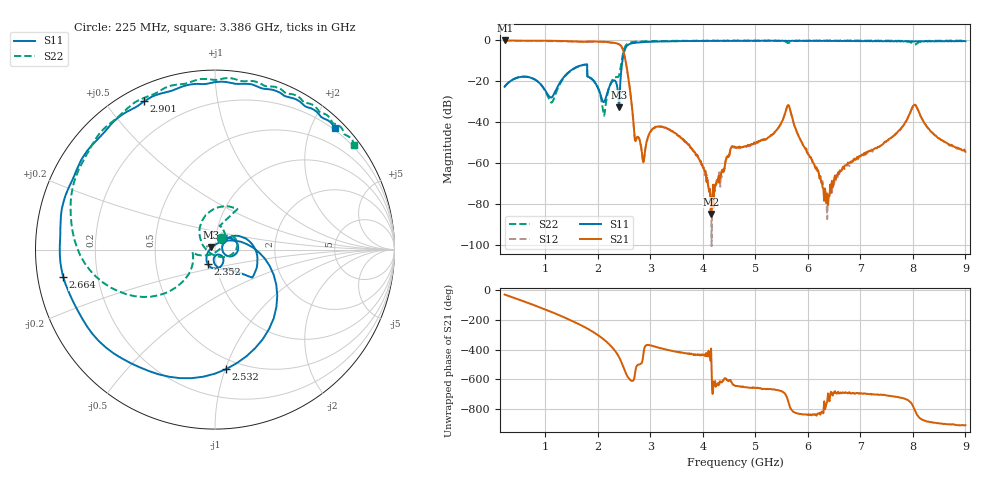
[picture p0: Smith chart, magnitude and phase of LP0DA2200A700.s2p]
!Agilent Technologies,E8358A,US41080443,A.07.50.56
!Agilent E8358A: A.07.50.56
!Date: Monday, May 09, 2016 11:42:41
!Correction: S11(Full 2 Port(1,2))
!S21(Full 2 Port(1,2))
!S12(Full 2 Port(1,2))
!S22(Full 2 Port(1,2))
!S2P File: Measurements: S11, S21, S12, S22:Log Frequency Sweep
# Hz S  dB  R 50
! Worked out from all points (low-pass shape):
!   1601 points, 225 MHz to 9 GHz, reference 50 ohm
!   highest |S21| = 0.00 dB at 226 MHz (marker M1); lowest = -85.0 dB at 4.157 GHz (marker M2)
!   |S21| within 3 dB of the highest: start of sweep to 2.452 GHz
!   lowest |S11| = -32.8 dB at 2.402 GHz (marker M3), VSWR 1.05, Z = 48.1 + j1.13 ohm
!   |S11| at or under -10 dB: start of sweep to 2.469 GHz
!   |S22| runs from -36.9 to 0.0 dB; largest |S21 - S12| = 0.021
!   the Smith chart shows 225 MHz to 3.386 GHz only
!   S11 on the Smith chart (normalised r, x): 225 MHz: 1.08, +0.13; 2.352 GHz: 0.91, -0.15; 2.532 GHz: 0.42, -1.01; 2.664 GHz: 0.08, -0.09; 2.901 GHz: 0.06, +0.63; 3.386 GHz: 0.17, +2.38
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2.25e8  -22.69 56.2  -0.01 -28.7  -0.17 -28.6  -22.63 62.2
2.260399e8  -22.67 56.0  -0.00 -28.9  -0.17 -28.7  -22.59 62.2
8.748646e8  -20.51 -24.1  -0.14 -112.0  -0.31 -111.9  -20.49 -17.8
1.122225e9  -27.89 12.8  -0.16 -146.6  -0.34 -146.5  -30.40 -124.2
1.687749e9  -12.22 -15.6  -0.60 123.1  -0.77 123.1  -12.26 79.7
2.115602e9  -30.19 -68.5  -0.64 28.1  -0.82 28.2  -36.82 -49.7
2.352303e9  -20.85 -116.0  -1.37 -59.9  -1.54 -59.8  -17.94 -173.3
2.401623e9  -32.84 149.1  -1.80 -88.5  -1.96 -88.4  -17.23 -152.9
2.532412e9  -3.50 -84.6  -10.52 162.0  -10.64 161.9  -2.48 -177.5
2.664175e9  -1.32 -169.7  -35.93 109.6  -36.07 109.3  -0.77 130.5
2.901418e9  -0.77 115.5  -53.64 -17.0  -53.91 -16.7  -0.38 86.3
3.152512e9  -0.53 71.8  -42.16 -26.0  -42.19 -25.8  -0.28 57.2
3.386075e9  -0.44 45.4  -44.00 -45.9  -44.11 -46.7  -0.29 36.9
3.888426e9  -0.23 12.4  -55.95 -74.6  -56.22 -72.8  -0.13 6.5
4.157298e9  -0.23 1.5  -85.00 -33.0  -76.36 -69.6  -0.15 -5.2
4.622431e9  -0.25 -11.1  -52.24 74.3  -52.65 76.7  -0.13 -20.7
5.623152e9  -0.22 -27.3  -31.67 -25.9  -31.81 -25.8  -1.27 -43.0
6.081681e9  -0.19 -34.2  -58.56 -118.2  -59.08 -119.2  -0.09 -49.4
6.412882e9  -0.18 -40.4  -76.17 -28.0  -75.25 13.0  -0.04 -55.5
7.553438e9  -0.41 -73.3  -48.15 7.8  -48.49 8.0  -0.15 -77.9
8.038582e9  -0.43 -90.4  -31.43 -88.6  -31.60 -88.7  -2.05 -84.3
9e9  -0.37 -121.3  -54.54 171.1  -54.26 165.2  -0.13 -101.3
